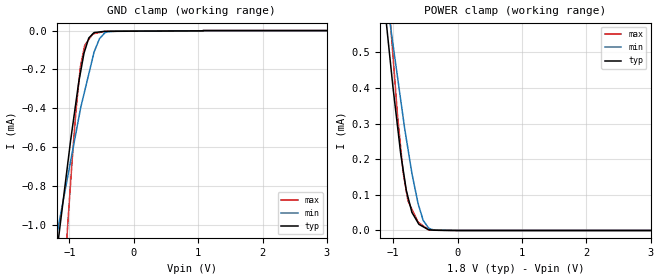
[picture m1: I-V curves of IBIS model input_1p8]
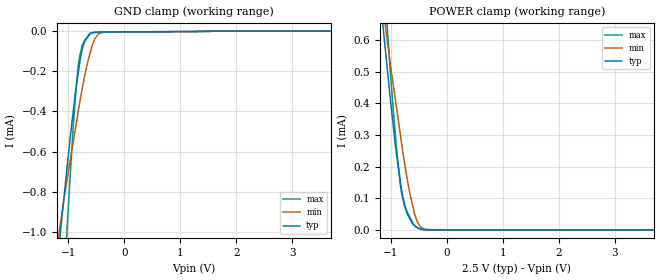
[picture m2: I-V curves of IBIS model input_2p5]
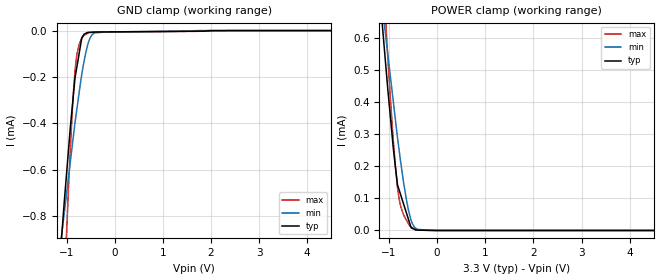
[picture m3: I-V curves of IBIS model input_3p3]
| Texas Instruments Incorporated
| ISO1042
| Marketing part#   Digital Voltage Range   Package-type   #pins
| ISO1042   1.71V - 5.5V   DW , DWV   16 , 8
[IBIS Ver]   4.1
[File name]   iso1044.ibs
[File Rev]   1.0
[Date]   12/14/2017
[Source]
| Texas Instruments Incorporated.
| Analog-eLab Design Center, HPA
| 12500 TI Blvd
| Dallas, TX -75243
[Notes]   Revision History:
| Rev 1.0: 12/14/2017
| - Initial version of the model
| - Model generated from simulations in SPECTRE
| - Model matched to SPICE simulation
| - C_comp although listed in numerical order of value are
|   obtained from varying PVT conditions. For PVT conditions for
|   each specific value refer the buffer description under
|   respective [Model]. IBIS model user is responsible for using
|   appropriate C_comp to simulate for Signal Integrity.
[Disclaimer]
| This model is designed as an aid for customers of Texas Instruments.
| TI and its licensors and suppliers make no warranties, either expressed
| or implied, with respect to this  model, including the warranties of
| merchantability or fitness for a particular purpose. The model is
| provided solely on an "as is" basis. The entire risk as to its quality
| and performance is with the customer.
[Copyright]
(C) Copyright 2017 Texas Instruments Incorporated.All rights reserved.
|   ISO1044
[Component]   ISO1044
[Manufacturer]   TI
[Package]   |8 D
|   typ   min   max
R_pkg   0.1   0.08   0.12
L_pkg   1.0nH   0.8nH   1.2nH
C_pkg   0.2pF   0.16pF   0.24pF
[Pin] signal_name  model_name   R_pin   L_pin   C_pin
1   VCC1   power   NA   NA   NA
2   TXD   input   NA   NA   NA
3   RXD   output   NA   NA   NA
4   GND1   gnd   NA   NA   NA
5   CANL   CANL   NA   NA   NA
6   CANH   CANH   NA   NA   NA
7   GND2   gnd   NA   NA   NA
8   VCC2   power   NA   NA   NA
|   Model Selectors
[Model Selector] input
input_1p8   1.8V   digital Input
input_2p5   2.5V   digital Input
input_3p3   3.3V   digital Input
input_5p0   5.0V   digital Input
[Model Selector] output
output_1p8   1.8V   digital Output
output_2p5   2.5V   digital Output
output_3p3   3.3V   digital Output
output_5p0   5.0V   digital Output
| Models and submodels in the file (10): input_1p8 (Input), input_2p5 (Input), input_3p3 (Input), input_5p0 (Input), output_1p8 (3-state), output_2p5 (3-state), output_3p3 (3-state), output_5p0 (3-state), CANH (I/O_open_source), CANL (I/O_open_drain)
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|   input_1p8 Model
[Model]   input_1p8
Model_type   Input
Vinl = 0.54
Vinh = 1.26
|   typ   min   max
C_comp   0.0009pF   0.0008pF   0.0142pF
|  Where Nom  PVT is Nominal Process, 1.8V,   27C
|   Fast PVT is Strong Process,  1.89V, -40C
|   Slow PVT is Weak Process,   1.71V,  150C
[Model spec]
|subparameter
Vinl   0.54   0.513   0.567
Vinh   1.26   1.197   1.323
[Voltage Range]   1.8   1.71   1.89
|Junction Temperature
[Temperature Range]   27   150   -40
[Power Clamp Reference]   1.8   1.71   1.89
[GND Clamp Reference]   0   0   0
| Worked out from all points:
|   GND clamp passes 1 mA (typ) near -1.14 V on its own axis
|   POWER clamp passes 1 mA (typ) near -1.33 V on its own axis
[GND Clamp]
|   Voltage   I(typ)   I(min)   I(max)
-1.8V     -2.881mA   -2.198mA   -5.365mA
-1.187V   -1.122mA   -1.037mA   -1.848mA
-1.169V   -1.071mA   -1.005mA   -1.754mA
-1.026V   -687.7uA   -753.4uA   -1.002mA
-898.1mV  -368.7uA   -527.1uA   -413.3uA
-828.8mV  -218uA     -404.8uA   -184.9uA
-761.5mV  -104.1uA   -310.4uA   -75.93uA
-699.2mV  -38.41uA   -224.4uA   -46.64uA
-616.9mV  -10.27uA   -111uA     -15.85uA
-533.6mV  -7.048uA   -42.48uA   -9.982uA
-387.9mV  -3.624uA   -5.553uA   -3.886uA
3.6V      0A         0A         0A
[POWER Clamp]
|   Voltage   I(typ)   I(min)   I(max)
-1.8V     1.875mA    1.62mA     2.877mA
-1.18V    713.4uA    754.1uA    966.4uA
-1.056V   495.3uA    592.1uA    617.4uA
-1.004V   404.9uA    525uA      494.9uA
-932.8mV  293.7uA    431.8uA    325.1uA
-846.4mV  172.7uA    319.4uA    165.1uA
-770.2mV  94.54uA    229.4uA    83.3uA
-708.7mV  50.84uA    160.9uA    59.86uA
-598.8mV  17.13uA    67.12uA    21.55uA
-533.5mV  10.52uA    28.43uA    12.9uA
-345.1mV  695.2nA    1.301uA    647.2nA
3.6V      0A         0A         0A
|   input_2p5 Model
[Model]   input_2p5
Model_type   Input
Vinl = 0.75
Vinh = 1.75
|   typ   min   max
C_comp   0.001pF   0.0008pF   0.0153pF
|  Where Nom  PVT is Nominal Process, 2.5V,   27C
|   Fast PVT is Strong Process,  2.75V, -40C
|   Slow PVT is Weak Process,   2.25V, 150C
[Model spec]
|subparameter
Vinl   0.75   0.675   0.825
Vinh   1.75   1.575   1.925
[Voltage Range]   2.5   2.25   2.75
|Junction Temperature
[Temperature Range]   27   150   -40
[Power Clamp Reference]   2.5   2.25   2.75
[GND Clamp Reference]   0   0   0
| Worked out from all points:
|   GND clamp passes 1 mA (typ) near -1.14 V on its own axis
|   POWER clamp passes 1 mA (typ) near -1.34 V on its own axis
[GND Clamp]
|   Voltage   I(typ)   I(min)   I(max)
-2.5V     -4.944mA   -3.557mA   -9.512mA
-1.223V   -1.223mA   -1.108mA   -2.04mA
-1.107V   -906.1uA   -892uA     -1.417mA
-1.023V   -674.6uA   -738.2uA   -985.1uA
-916.3mV  -407.3uA   -556.8uA   -488.3uA
-828.4mV  -218.1uA   -408.6uA   -184.7uA
-751.2mV  -89.47uA   -284.5uA   -68.07uA
-710.4mV  -47.12uA   -225.1uA   -52.21uA
-614mV    -10.94uA   -112.1uA   -14.74uA
-518.9mV  -6.058uA   -34.97uA   -7.082uA
-364.8mV  -4.789uA   -5.738uA   -5.294uA
5V        0A         0A         0A
[POWER Clamp]
|   Voltage   I(typ)   I(min)   I(max)
-2.5V     3.221mA    2.62mA     5.104mA
-1.196V   741.9uA    779.1uA    1.013mA
-1.079V   534.7uA    616.9uA    680.7uA
-1.062V   505.5uA    595uA      633.9uA
-967.6mV  344.8uA    472.4uA    401.9uA
-903.3mV  245.3uA    392.1uA    264.6uA
-804.7mV  121.8uA    269.1uA    112.4uA
-710.4mV  51.69uA    162.8uA    57.76uA
-576.8mV  13.43uA    50.81uA    15.28uA
-523.1mV  6.454uA    24.5uA     6.671uA
-298.1mV  682nA      775.6nA    524nA
5V        0A         0A         0A
|   input_3p3 Model
[Model]   input_3p3
Model_type   Input
Vinl = 0.99
Vinh = 2.31
|   typ   min   max
C_comp   0.001pF   0.0008pF   0.0163pF
|  Where Nom  PVT is Nominal Process, 3.3V,   27C
|   Fast PVT is Strong Process,  3.0V,  -40C
|   Slow PVT is Weak Process,   3.6V,   150C
[Model spec]
|subparameter
Vinl   0.99   0.9   1.08
Vinh   2.31   2.1   2.52
[Voltage Range]   3.3   3   3.6
|Junction Temperature
[Temperature Range]   27   150   -40
[Power Clamp Reference]   3.3   3   3.6
[GND Clamp Reference]   0   0   0
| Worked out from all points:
|   GND clamp passes 1 mA (typ) near -1.14 V on its own axis
|   POWER clamp passes 1 mA (typ) near -1.34 V on its own axis
[GND Clamp]
|   Voltage   I(typ)   I(min)   I(max)
-3.3V     -7.323mA   -5.124mA   -14.29mA
-1.124V   -949uA     -920.7uA   -1.512mA
-1.047V   -740.3uA   -787.5uA   -1.115mA
-1.018V   -664.4uA   -735.4uA   -959.9uA
-955.7mV  -506.2uA   -627uA     -663.2uA
-862.5mV  -288uA     -463.9uA   -284uA
-804.1mV  -180.1uA   -367uA     -133.7uA
-682.5mV  -30.8uA    -189.1uA   -33uA
-560.9mV  -8.079uA   -62.44uA   -11.34uA
-415mV    -6.331uA   -9.499uA   -7.565uA
-113mV    -5.638uA   -5.726uA   -6.303uA
6.6V      0A         0A         0A
[POWER Clamp]
|   Voltage   I(typ)   I(min)   I(max)
-3.3V     4.773mA    3.773mA    7.668mA
-1.151V   661.5uA    714.9uA    878.3uA
-1.121V   608.3uA    673.2uA    796.6uA
-1.032V   451.5uA    558.4uA    555.6uA
-913.4mV  260.3uA    405.3uA    284.8uA
-825mV    142.9uA    290.9uA    135.7uA
-797.7mV  130uA      259.3uA    105.5uA
-738.4mV  102uA      192.7uA    65.75uA
-596.9mV  35.09uA    63.89uA    21.19uA
-540.1mV  8.254uA    31.32uA    10.73uA
-446.7mV  1.993uA    7.311uA    1.722uA
6.6V      0A         0A         0A
